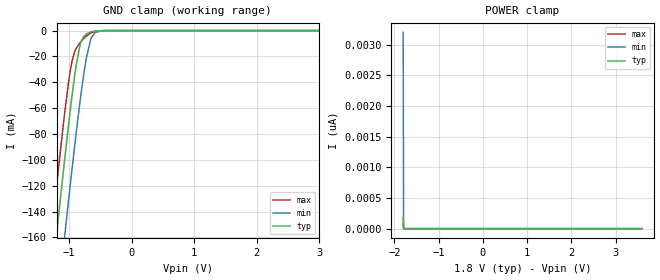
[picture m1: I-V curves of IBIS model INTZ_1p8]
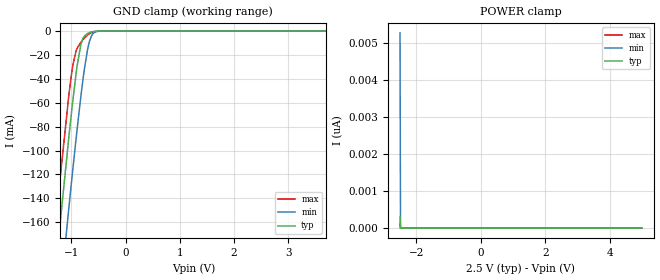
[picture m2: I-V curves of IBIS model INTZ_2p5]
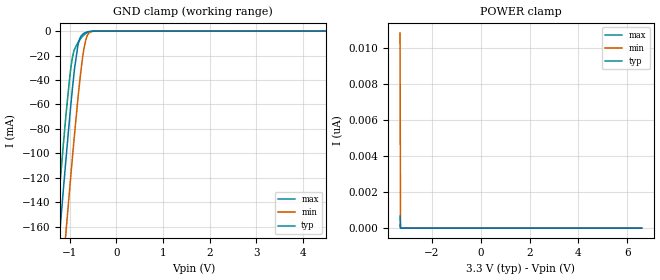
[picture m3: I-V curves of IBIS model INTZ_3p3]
|Texas Instruments Incorporated
| Low Voltage 4-Channel I2C and SMBus Switch with Reset Function
| part#   Digital Voltage Range   Package-type   #pins
| TCA9546A   1.65V - 5.5V   TSSOP   16
[IBIS Ver]   4.1
[File name]   tca9546a.ibs
[File Rev]   1.0
[Date]   04/02/2014
[Source]
| Texas Instruments Incorporated.
| 12500 TI Blvd
| Dallas, TX -75243
[Notes]   Revision History:
| Rev 1.0: 04/02/2014
| - Initial version of the model
| - Model generated from simulations in TISPICE
| - C_comp although listed in numerical order of value are
|   obtained from varying PVT conditions. For PVT conditions for
|   each specific value refer the buffer description under
|   respective [Model]. IBIS model user is responsible for using
|   appropriate C_comp to simulate for Signal Integrity.
| - Warnings regarding combined/Non-monotonicity of various models have been
|   reviewd and considered minor and can be ignored.
| - Model names with a trailing _1p8 contains the model for 1.8V operation.
|   Model names with a trailing _2p5 contains the model for 2.5V operation.
|   Model names with a trailing _3p3 contains the model for 3.3V operation.
|   Model names with a trailing _5p0 contains the model for 5.0V operation.
[Disclaimer]
| This model is designed as an aid for customers of Texas Instruments.
| TI and its licensors and suppliers make no warranties, either expressed
| or implied, with respect to this  model, including the warranties of
| merchantability or fitness for a particular purpose. The model is
| provided solely on an "as is" basis. The entire risk as to its quality
| and performance is with the customer.
[Copyright]
 (C) Copyright 2014 Texas Instruments Incorporated.All rights reserved.
|   Device
[Component]   TCA9546A
[Manufacturer]   TI
[Package]
|   typ   min   max
R_pkg   0.1347   0.1220   0.1466
L_pkg   2.8895nH 2.4371nH   3.3817nH
C_pkg   0.4678pF   0.4043pF  0.5383pF
[Pin]  signal_name   model_name   R_pin   L_pin   C_pin
1   A0   INTZ   0.13944   3.38172nH   0.52364pF
2   A1   INTZ   0.14662   3.15427nH   0.53825pF
3   RESETB   INTZ   0.13206   2.59919nH   0.4043pF
4   SD0   NC   0.12293   2.45188nH   0.40645pF
5   SC0   NC   0.12301   2.45516nH   0.40656pF
6   SD1   NC   0.13227   2.60697nH   0.40606pF
7   SC1   NC   0.14089   3.06601nH   0.5301pF
8   GND   GND   0.13768   3.36289nH   0.51785pF
9   SD2   NC   0.13409   3.30669nH   0.51775pF
10   SC2   NC   0.14519   3.13431nH   0.53537pF
11   SD3   NC   0.13867   2.70837nH   0.41301pF
12   SC3   NC   0.12446   2.47816nH   0.41058pF
13   A2   INTZ   0.12196   2.43708nH   0.40806pF
14   SCL   SCL   0.13191   2.59669nH   0.40679pF
15   SDA   SDA   0.14417   3.11547nH   0.53595pF
16   VCC   POWER   0.13915   3.37722nH   0.52339pF
|   Model Selectors
[Model Selector]  SDA
SDA_5p0   SDA buffer at 5.0V operation
SDA_3p3   SDA buffer at 3.3V operation
SDA_2p5   SDA buffer at 2.5V operation
SDA_1p8   SDA buffer at 1.8V operation
[Model Selector]  SCL
SCL_5p0   SCL buffer at 5.0V operation
SCL_3p3   SCL buffer at 3.3V operation
SCL_2p5   SCL buffer at 2.5V operation
SCL_1p8   SCL buffer at 1.8V operation
[Model Selector]  INTZ
INTZ_5p0   Input buffer at 5.0V operation
INTZ_3p3   Input buffer at 3.3V operation
INTZ_2p5   Input buffer at 2.5V operation
INTZ_1p8   Input buffer at 1.8V operation
| Models and submodels in the file (12): INTZ_1p8 (Input), INTZ_2p5 (Input), INTZ_3p3 (Input), INTZ_5p0 (Input), SCL_1p8 (Input), SCL_2p5 (Input), SCL_3p3 (Input), SCL_5p0 (Input), SDA_1p8 (I/O_open_drain), SDA_2p5 (I/O_open_drain), SDA_3p3 (I/O_open_drain), SDA_5p0 (I/O_open_drain)
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|   Model
[Model]   INTZ_1p8
Model_type   Input
Vinl = 0.54
Vinh = 1.26
|   typ   min   max
C_comp   1.378pF   1.292pF   1.466pF
[Voltage Range]   1.8   1.65   1.95
[Temperature Range]   27   125   -40
[Power Clamp Reference]   1.8   1.65   1.95
[GND Clamp Reference]   -0   -0   -0
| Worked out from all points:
|   GND clamp passes 1 mA (typ) near -0.65 V on its own axis
[GND Clamp]
|   Voltage   I(typ)   I(min)   I(max)
-1.8V     -444.5mA   -504.4mA   -407.1mA
-1.438V   -270.2mA   -330.8mA   -232.3mA
-1.222V   -168.5mA   -229.1mA   -130.8mA
-1.184V   -151.1mA   -211.6mA   -113.6mA
-1.071V   -100.1mA   -159.8mA   -64.28mA
-968.4mV  -56.83mA   -114.3mA   -27.68mA
-887.4mV  -27.43mA   -79.99mA   -13.89mA
-811.8mV  -9.407mA   -50.31mA   -8.666mA
-725.4mV  -2.729mA   -21.86mA   -4.347mA
-644.4mV  -935.9uA   -5.718mA   -1.642mA
-450mV    -25.03uA   -60uA      -30.72uA
3.595V    0A         0A         0A
[POWER Clamp]
|   Voltage   I(typ)   I(min)   I(max)
-1.8V     179.4pA    3.2nA      72.27pA
-1.789V   0A         0A         0A
-1.784V   0A         0A         0A
3.595V    0A         0A         0A
|   Model
[Model]   INTZ_2p5
Model_type   Input
Vinl = 0.75
Vinh = 1.75
|   typ   min   max
C_comp   1.378pF   1.292pF   1.466pF
[Voltage Range]   2.5   2.3   2.7
[Temperature Range]   27   125   -40
[Power Clamp Reference]   2.5   2.3   2.7
[GND Clamp Reference]   -0   -0   -0
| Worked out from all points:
|   GND clamp passes 1 mA (typ) near -0.65 V on its own axis
[GND Clamp]
|   Voltage   I(typ)   I(min)   I(max)
-2.5V     -787mA     -845.5mA   -750.7mA
-1.48V    -290.1mA   -350.6mA   -252.3mA
-1.285V   -197.8mA   -258.4mA   -159.9mA
-1.218V   -166.4mA   -226.9mA   -128.7mA
-1.052V   -92.02mA   -151.4mA   -56.8mA
-970mV    -57.47mA   -115mA     -28.12mA
-910mV    -34.93mA   -89.36mA   -16.29mA
-827.5mV  -12.06mA   -56.22mA   -9.593mA
-692.5mV  -1.8mA     -13.74mA   -3.073mA
-610mV    -552.2uA   -2.69mA    -947uA
-475mV    -43.19uA   -107.4uA   -55.89uA
4.992V    0A         0A         0A
[POWER Clamp]
|   Voltage   I(typ)   I(min)   I(max)
-2.5V     306.4pA    5.259nA    105.1pA
-2.485V   0A         0A         0A
-2.478V   0A         0A         0A
4.992V    0A         0A         0A
|   Model
[Model]   INTZ_3p3
Model_type   Input
Vinl = 0.99
Vinh = 2.31
|   typ   min   max
C_comp   1.378pF   1.292pF   1.466pF
[Voltage Range]   3.3   3   3.6
[Temperature Range]   27   125   -40
[Power Clamp Reference]   3.3   3   3.6
[GND Clamp Reference]   -0   -0   -0
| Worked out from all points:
|   GND clamp passes 1 mA (typ) near -0.65 V on its own axis
[GND Clamp]
|   Voltage   I(typ)   I(min)   I(max)
-3.3V     -1.182A    -1.239A    -1.146A
-1.34V    -223.5mA   -284.2mA   -185.6mA
-1.28V    -195.6mA   -256.3mA   -157.7mA
-1.211V   -163.4mA   -223.9mA   -125.7mA
-1.082V   -105.1mA   -164.9mA   -69mA
-943.8mV  -47.25mA   -103.7mA   -21.79mA
-825mV    -11.6mA    -55.27mA   -9.442mA
-735.9mV  -3.119mA   -24.84mA   -4.801mA
-656.7mV  -1.116mA   -7.317mA   -1.956mA
-577.5mV  -319uA     -1.25mA    -520.2uA
-409.2mV  -9.659uA   -23.55uA   -10.74uA
6.59V     0A         0A         0A
[POWER Clamp]
|   Voltage   I(typ)   I(min)   I(max)
-3.3V     664pA      10.84nA    162.7pA
-3.28V    0A         0A         0A
-3.27V    0A         0A         0A
6.59V     0A         0A         0A
